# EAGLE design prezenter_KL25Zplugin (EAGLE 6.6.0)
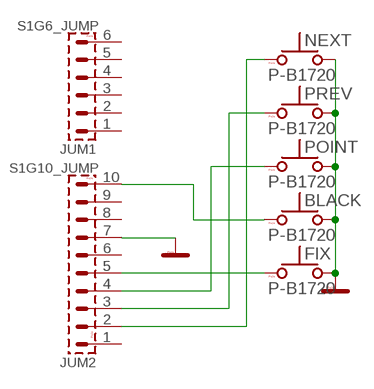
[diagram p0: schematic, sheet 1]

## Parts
BLACK  P-B1720  [P-B1720]
FIX  P-B1720  [P-B1720]
JUM1  S1G6_JUMP  [S1G6_JUM]
JUM2  S1G10_JUMP  [S1G10_JU]
NEXT  P-B1720  [P-B1720]
POINT  P-B1720  [P-B1720]
PREV  P-B1720  [P-B1720]

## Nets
GND: BLACK.3 FIX.3 JUM2.7 NEXT.3 POINT.3 PREV.3
N$1: JUM2.2 NEXT.1
N$2: JUM2.3 PREV.1
N$3: JUM2.4 POINT.1
N$4: FIX.1 JUM2.5
N$5: BLACK.1 JUM2.10
Unconnected: BLACK.2(1A) BLACK.4(2A) FIX.2(1A) FIX.4(2A) JUM1.1 JUM1.2 JUM1.3 JUM1.4 JUM1.5 JUM1.6 JUM2.1 JUM2.6 JUM2.8 JUM2.9 NEXT.2(1A) NEXT.4(2A) POINT.2(1A) POINT.4(2A) PREV.2(1A) PREV.4(2A)

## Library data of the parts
BLACK FIX NEXT POINT PREV = #PaJa_prepinace:P-B1720: &micro;-tlacitko
JUM1 = #PaJa_konektory:S1G6_JUMP: Radove konektory - koliky - 6x
JUM2 = #PaJa_konektory:S1G10_JUMP: Radove konektory - koliky - 10x

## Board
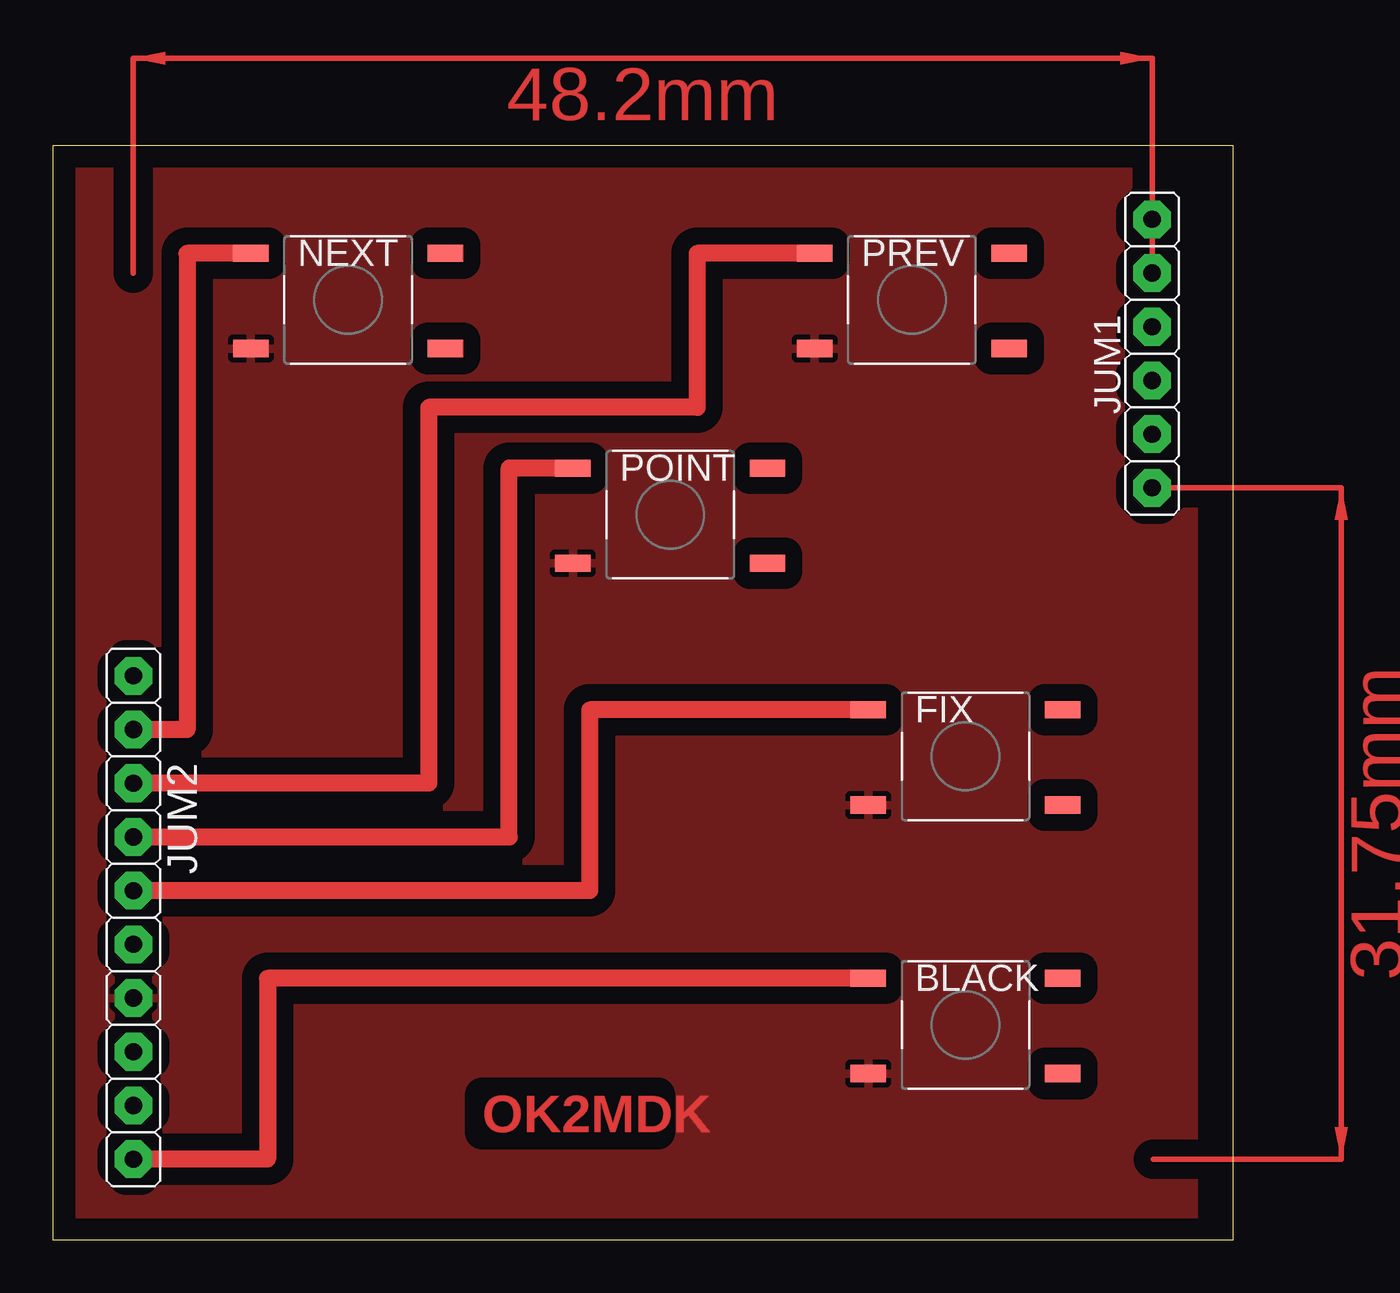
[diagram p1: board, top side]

Size 55.86 x 51.74 mm. Coordinates in mm from the lower left corner, seen from the top.
Outline: 0,0 55.86,0 55.86,51.74 0,51.74 0,0
Copper layers (1*16): Top 0.035mm / dielectric 1.5mm / Bottom 0.035mm
Design rules "default": minimum track width 10mil, minimum drill 24mil, track to track 8mil, track to pad 8mil, pad to pad 8mil, via to via 8mil, smd to smd 8mil, copper to edge 40mil, drill to drill 8mil, minimum pad ring 10mil, minimum via ring 8mil, stop-mask expansion 4mil, vias tented up to drill 0mil, thermal gap 10mil

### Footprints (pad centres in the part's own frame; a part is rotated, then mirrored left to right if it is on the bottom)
P-B1720 = smd 1.676 x 0.813: 1 -4.6,2.2; 2 4.6,2.2; 3 -4.6,-2.3; 4 4.6,-2.3
S1G6_JUM = drill 0.813 pad 1.778 octagon: 1 -6.35,0; 2 -3.81,0; 3 -1.27,0; 4 1.27,0; 5 3.81,0; 6 6.35,0
S1G10_JU = drill 0.813 pad 1.778 octagon: 1 -11.43,0; 2 -8.89,0; 3 -6.35,0; 4 -3.81,0; 5 -1.27,0; 6 1.27,0; 7 3.81,0; 8 6.35,0; 9 8.89,0; 10 11.43,0

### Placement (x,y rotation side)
BLACK  43.18,10.16 0 top
FIX  43.18,22.86 0 top
JUM1  52.01,41.91 90 top
JUM2  3.81,15.24 270 top
NEXT  13.97,44.45 0 top
POINT  29.21,34.29 0 top
PREV  40.64,44.45 0 top

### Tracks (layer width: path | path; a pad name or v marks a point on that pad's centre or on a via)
GND
  pour Top (isolate 0.813): 1.27,0 53.98,0 53.98,50.8 1.27,50.8
N$1
  Top 0.813: NEXT.1 6.35,46.65 6.35,24.13 JUM2.2
N$2
  Top 0.813: PREV.1 30.48,46.65 30.48,39.37 17.78,39.37 17.78,21.59 JUM2.3
N$3
  Top 0.813: JUM2.4 21.59,19.05 21.59,36.49 POINT.1
N$4
  Top 0.813: FIX.1 25.4,25.06 25.4,16.51 JUM2.5
N$5
  Top 0.813: BLACK.1 10.16,12.36 10.16,3.81 JUM2.10
(copper drawn outside any net)
  shapes: Top area x2

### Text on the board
Top: OK2MDK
